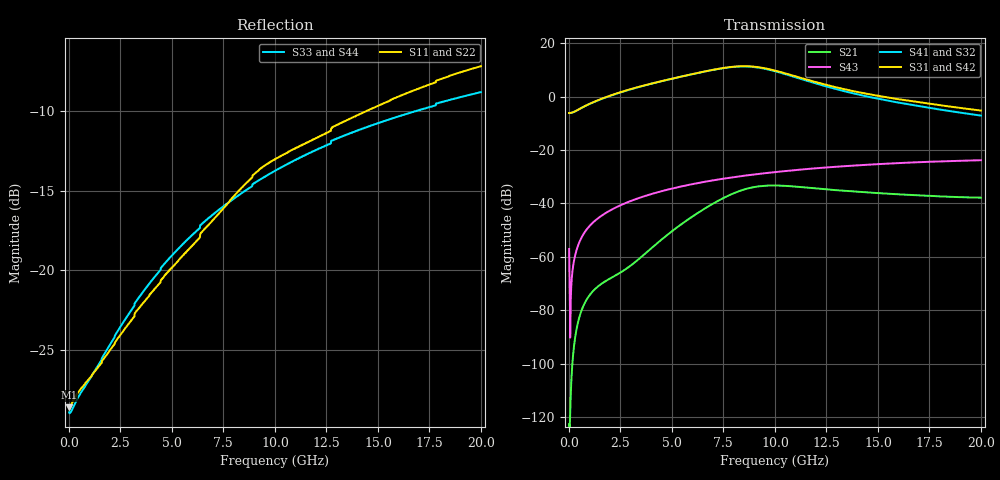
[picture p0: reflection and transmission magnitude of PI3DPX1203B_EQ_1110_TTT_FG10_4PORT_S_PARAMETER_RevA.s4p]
! NPort=4 DATA=2000 NOISE=0 GROUPDELAY=0 COMPLEX_DATAFORMAT=POLAR
! NumOfBlock=1 NumOfParam=0
! .MODEL Smodel S TSTONEFILE=PI3DPX1203B_EQ_1110_TTT_FG10_4PORT_S_PARAMETER_RevA.s4p TYPE=S
!  -- The above .MODEL line can be used for the S element in the netlist.
! The s parameter is extracted from the linear redriver, it is not bi-directional; only s(4,1)s(4,2) and s(3,1)s(3,2)
! should be the insertion loss
!Port definition:
!Port1 = input+
!Port2 = input-
!Port3 = output+
!Port4 = output-
# Hz S MA R  50
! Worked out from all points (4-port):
!   2000 points, 10 MHz to 20 GHz, reference 50 ohm
!   strongest paths, dB at 10 MHz, 5.01 GHz, 10.01 GHz, 15.01 GHz, 20 GHz:
!     S31: -6.2, 6.7, 9.7, 0.3, -5.2
!     S42: -6.2, 6.7, 9.7, 0.3, -5.2
!     S41: -6.2, 6.7, 9.5, -0.8, -7.1
!     S32: -6.2, 6.7, 9.5, -0.8, -7.1
!     S43: -57.1, -34.4, -28.3, -25.3, -23.8
!     S21: -122.7, -50.4, -33.3, -36.1, -37.9
!   lowest |S11| = -28.6 dB at 10 MHz (marker M1), VSWR 1.08, Z = 46.4 - j0.0306 ohm
!   |S11| at or under -10 dB: start of sweep to 14.41 GHz
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1e7  0.03701 -179.5  7.338e-07 10.7  0 0.0  0 0.0
     7.338e-07 10.7  0.03701 -179.5  0 0.0  0 0.0
     0.4917 0.0  0.4917 -180.0  0.03566 178.2  0.001403 -77.8
     0.4917 -180.0  0.4917 0.0  0.001403 -77.8  0.03566 178.2
3e9  0.06913 -127.5  0.0006855 146.8  1.245e-10 58.0  2.226e-09 108.1
     0.0006854 146.8  0.06913 -127.5  2.226e-09 108.1  1.245e-10 58.0
     1.38 5.1  1.368 -173.8  0.07437 -127.1  0.01108 78.0
     1.368 -173.8  1.38 5.1  0.01108 78.0  0.07437 -127.1
5.66e9  0.1133 -111.2  0.004628 156.0  1.01e-08 -122.3  9.558e-08 71.0
        0.004627 156.0  0.1133 -111.2  9.555e-08 71.0  1.01e-08 -122.3
        2.469 -37.6  2.467 143.8  0.1231 -117.5  0.0216 66.7
        2.467 143.8  2.469 -37.6  0.0216 66.7  0.1231 -117.5
8.08e9  0.1731 -104.8  0.01593 111.3  2.761e-07 155.2  7.779e-07 21.4
        0.01593 111.4  0.1731 -104.8  7.772e-07 21.5  2.761e-07 155.3
        3.651 -98.2  3.618 82.9  0.1695 -115.8  0.03132 54.5
        3.619 82.9  3.65 -98.2  0.03132 54.5  0.1695 -115.8
9.66e9  0.2169 -107.3  0.02155 67.4  9.974e-07 94.3  1.692e-06 -16.3
        0.02153 67.4  0.2169 -107.3  1.69e-06 -16.2  9.977e-07 94.4
        3.299 -149.0  3.224 32.0  0.1998 -116.1  0.03726 46.1
        3.225 32.0  3.298 -149.0  0.03726 46.1  0.1998 -116.1
1.191e10  0.2589 -109.4  0.01924 26.5  2.76e-06 29.6  3.41e-06 -44.8
          0.01922 26.6  0.2589 -109.4  3.41e-06 -44.6  2.762e-06 29.6
          1.902 162.1  1.795 -16.8  0.2376 -117.4  0.04517 34.7
          1.796 -16.8  1.901 162.1  0.04517 34.7  0.2376 -117.4
2e10  0.4391 -117.8  0.01275 -18.1  2.243e-05 -109.9  3.109e-05 -133.8
      0.0128 -18.0  0.4392 -117.8  3.117e-05 -133.7  2.246e-05 -109.9
      0.5467 72.9  0.4406 -95.3  0.3637 -123.9  0.06431 -7.1
      0.4404 -95.4  0.5473 73.0  0.06431 -7.1  0.3637 -123.9
